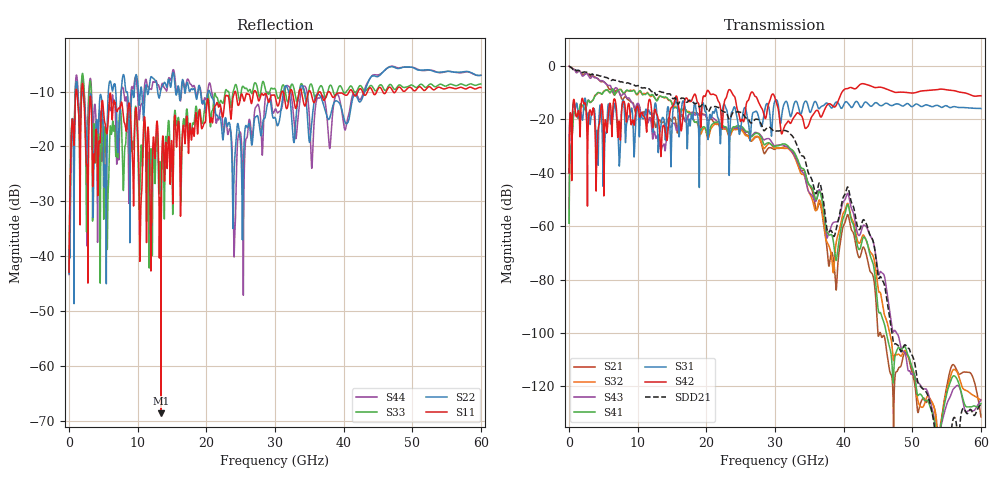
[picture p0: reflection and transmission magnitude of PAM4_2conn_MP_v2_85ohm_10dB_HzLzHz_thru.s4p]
! Info: Touchstone file created by Circ.  Input file=FAB50GbE_2conn_Midplane_Examax_Topo2_v2_85ohm_10dB_HzLzHz.circ
# Hz S RI R 50
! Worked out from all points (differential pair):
!   6000 points, 10 MHz to 60 GHz, reference 50 ohm
!   strongest paths, dB at 10 MHz, 15.01 GHz, 30.01 GHz, 45.01 GHz, 60 GHz:
!     S42: -40.1, -15.4, -12.0, -8.0, -11.2
!     S31: -40.2, -22.5, -13.0, -14.2, -15.9
!     S41: -58.9, -14.3, -30.2, -90.7, -126.4
!     S43: -0.1, -21.9, -29.9, -77.1, -125.1
!     S32: -58.9, -14.2, -30.8, -83.0, -125.1
!     S21: -0.1, -20.4, -31.2, -100.7, -131.4
!   taken as a pair (ports 3,1 in; 4,2 out), SDD21 dB: -0.1, -11.9, -24.6, -78.3, -126.7
!   lowest |S11| = -68.7 dB at 13.39 GHz (marker M1), VSWR 1.00, Z = 50 + j0.000912 ohm
!   |S11| at or under -10 dB: 2.109 GHz to 24.15 GHz (22.04 GHz wide, 168 % of centre); 27.22 GHz to 30.99 GHz (3.776 GHz wide, 13 % of centre); 37.9 GHz to 40.8 GHz (2.903 GHz wide, 7.38 % of centre)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
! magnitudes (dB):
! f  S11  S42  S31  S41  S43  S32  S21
! 10 MHz  -42.9  -40.1  -40.2  -58.9  -0.1  -58.9  -0.1
! 1.81 GHz  -10.5  -13.3  -18.6  -14.4  -3.3  -14.7  -2.7
! 13.39 GHz  -68.7  -33.9  -22.4  -11.4  -31.7  -11.4  -21.2
! 24.12 GHz  -10.1  -11.5  -15.4  -22.8  -23.3  -23.8  -23.5
! 32.29 GHz  -9.6  -21.5  -19.0  -31.1  -31.6  -31.8  -31.3
! 38.42 GHz  -11.0  -15.0  -15.4  -64.5  -58.8  -76.0  -70.9
! 60 GHz  -9.2  -11.2  -15.9  -126.4  -125.1  -125.1  -131.4
